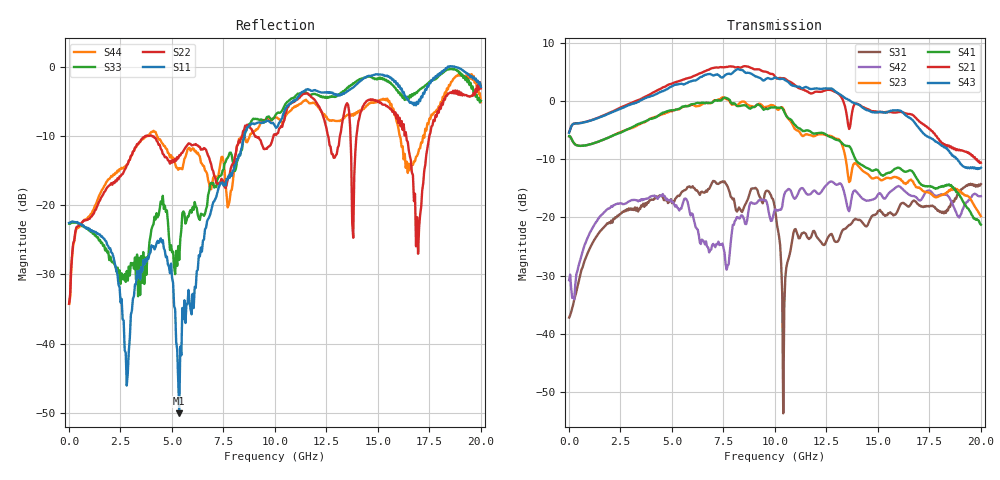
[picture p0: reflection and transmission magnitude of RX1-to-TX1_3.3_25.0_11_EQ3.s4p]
!Agilent Technologies,N5225A,MY51451112,A.09.50.13
!Agilent N5225A: A.09.50.13
!Date: Wednesday, January 31, 2018 11:03:14
!Correction: S11(Full 4 Port(1,2,3,4))
!S12(Full 4 Port(1,2,3,4))
!S13(Full 4 Port(1,2,3,4))
!S14(Full 4 Port(1,2,3,4))
!S21(Full 4 Port(1,2,3,4))
!S22(Full 4 Port(1,2,3,4))
!S23(Full 4 Port(1,2,3,4))
!S24(Full 4 Port(1,2,3,4))
!S31(Full 4 Port(1,2,3,4))
!S32(Full 4 Port(1,2,3,4))
!S33(Full 4 Port(1,2,3,4))
!S34(Full 4 Port(1,2,3,4))
!S41(Full 4 Port(1,2,3,4))
!S42(Full 4 Port(1,2,3,4))
!S43(Full 4 Port(1,2,3,4))
!S44(Full 4 Port(1,2,3,4))
!S4P File: Measurements: <S11,S12,S13,S14>,
!<S21,S22,S23,S24>,
!<S31,S32,S33,S34>,
!<S41,S42,S43,S44>:
# Hz S  RI  R 50
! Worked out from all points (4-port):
!   401 points, 10 MHz to 20 GHz, reference 50 ohm
!   strongest paths, dB at 10 MHz, 5.008 GHz, 10.01 GHz, 15 GHz, 20 GHz:
!     S43: -5.5, 2.5, 4.0, -1.9, -11.5
!     S21: -5.4, 3.0, 4.2, -1.9, -10.6
!     S41: -6.1, -1.6, -1.1, -11.9, -21.2
!     S23: -6.1, -1.8, -0.9, -13.2, -19.8
!     S42: -30.8, -17.3, -18.6, -16.1, -16.3
!     S31: -37.2, -17.5, -18.5, -18.9, -14.3
!   lowest |S11| = -50.1 dB at 5.357 GHz (marker M1), VSWR 1.01, Z = 50.3 - j0.157 ohm
!   |S11| at or under -10 dB: start of sweep to 8.517 GHz
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1e7  -0.0744 -0.00329  -0.000651 0.00034  0.0136 0.000522  -0.000387 0.000347
     0.5364 0.00778  -0.0133 0.0143  -0.4977 0.00393  0.0263 0.0121
     0.0138 0.000389  -6.02e-06 0.000246  -0.0734 -0.00402  -0.000243 0.000328
     -0.4977 0.0039  0.0264 0.0119  0.5338 0.0075  -0.0128 0.0145
5.357325e9  0.00272 -0.00156  0.0291 -0.005  0.0866 0.1386  0.0287 -0.0143
            -0.6656 -1.324  0.1296 -0.1893  0.5544 0.6412  0.1175 0.0114
            0.0811 0.1295  0.0347 -0.00114  0.0352 0.0195  0.0389 -0.0131
            0.7277 0.4505  0.1132 0.0194  -1.067 -0.9015  0.068 -0.1723
7.2064e9  -0.0226 0.121  0.0158 -0.0199  0.1308 0.0977  0.0019 -0.0303
          -1.928 0.1283  0.1305 -0.0594  0.9774 -0.2815  0.0588 0.0249
          0.1581 0.1132  0.0227 -0.0274  0.0106 0.1535  0.00513 -0.0432
          0.7543 -0.6625  0.0589 -0.000751  -1.42 0.9187  0.1204 -0.097
8.855575e9  0.0105 0.388  0.0122 -0.0168  0.1295 0.1009  -0.00587 -0.0155
            -0.5948 1.821  -0.1008 0.3417  0.1477 -0.8906  0.0342 0.1217
            0.1446 0.1019  0.00114 -0.0216  0.0626 0.3989  -0.0138 -0.0236
            -0.2447 -0.834  0.0172 0.1339  0.4215 1.66  0.2692 0.1871
1.275362e10  0.2739 0.5853  -0.0384 -0.00659  0.0264 0.0598  -0.0319 0.0101
             1.107 -0.5473  0.164 0.1676  -0.4171 0.2718  0.1904 0.105
             0.03 0.0658  -0.0308 -0.00838  0.4054 0.4604  -0.0436 0.00157
             -0.1611 0.4589  0.178 0.0977  0.373 -1.22  0.2176 -0.3439
1.665168e10  0.5254 0.1375  -0.0278 0.0163  -0.0608 0.1092  -0.00303 0.0373
             -0.6681 -0.3704  0.00808 0.1719  0.1033 0.1792  0.0945 0.1095
             -0.0654 0.1183  -0.026 0.00427  0.6081 -0.1765  -0.00836 0.037
             0.2504 0.00206  0.1082 0.1083  -0.4992 0.4804  -0.1106 -0.1611
2e10  0.7136 0.0598  0.023 0.0349  -0.0797 0.1691  0.0344 0.0208
      -0.0656 0.2877  0.6931 0.0766  0.0929 -0.0438  0.1512 0.0434
      -0.0825 0.1745  0.00632 0.0477  0.5676 -0.031  0.0478 0.0206
      -0.0121 -0.086  0.1454 0.0458  0.2192 0.1527  -0.1526 -0.5341
